(* Logix 5000 Rung export; software revision 16.04 *)

TYPE SIEDATETIME :   // Stores the date and time value
STRUCT
   Year : DINT;   // Displays module current year
   Month : DINT;   // Displays Module current month
   Day : DINT;   // Displays Module current day
   Hour : DINT;   // Displays Module current hour
   Minute : DINT;   // Displays Module current minute
   Seconds : DINT;   // Displays Module current second
END_STRUCT
END_TYPE

TYPE SIEETHERNETTYPE :   // Allows read/write Ethernet settings between the module and processor
STRUCT
   Read : BOOL;   // Enable Ethernet configuration transfer from module to processor
   Write : BOOL;   // Enable Ethernet configuration transfer from processor to module
   Config : SIEETHERNET;   // Module ethernet configurations ip, netmask and gateway
END_STRUCT
END_TYPE

TYPE SIEETHERNET :   // Stores the MVI56E-SIE IP settings
STRUCT
   IP : INT[4];   // Module IP address
   Netmask : INT[4];   // Net mask used by the Module
   Gateway : INT[4];   // Gateway used by the module
END_STRUCT
END_TYPE

TYPE SIECLOCKTYPE :   // Allows read/write of clock value between the module and processor
STRUCT
   Read : BOOL;   // Reads current time from the module
   Write : BOOL;   // Writes current time from the module
   Config : SIEDATETIME;   // Date and time configuration read or written between the module and processor
END_STRUCT
END_TYPE

ADD_ON_INSTRUCTION AOI56ESIE_OPTIONAL   (* revision 1.0 *)
// MVI56E-SIEOptional Add-On Ethernet/Clock
// Revision note:
// Release
VAR_IN_OUT
   MVI56SIEEthernet : SIEETHERNETTYPE; {required}   // MVI56E-SIE Rev2 Ethernet Settings
        .READ   // MVI56E-SIE Rev2 Ethernet Settings Enable Ethernet configuration transfer from module to processor
   MVI56SIEClock : SIECLOCKTYPE; {required}   // MVI56E-SIE Rev2 Clock Settings
   ReadEthernetMSG : MESSAGE; {required}   // Read Ethernet Settings Message
   WriteEthernetMSG : MESSAGE; {required}   // Write Ethernet Settings Message
   ReadClockMSG : MESSAGE; {required}   // Read Clock Settings Message
   WriteClockMSG : MESSAGE; {required}   // Write Clock Settings Message
END_VAR

ROUTINE Logic   (* ladder *)
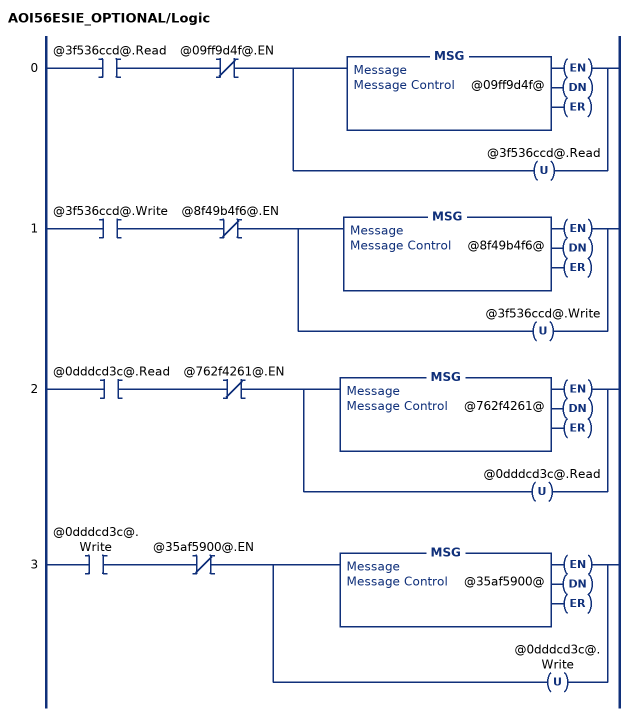
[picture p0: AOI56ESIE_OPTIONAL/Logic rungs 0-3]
   0: XIC(@3f536ccd@.Read)XIO(@09ff9d4f@.EN)[MSG(@09ff9d4f@) ,OTU(@3f536ccd@.Read) ];
   1: XIC(@3f536ccd@.Write)XIO(@8f49b4f6@.EN)[MSG(@8f49b4f6@) ,OTU(@3f536ccd@.Write) ];
   2: XIC(@0dddcd3c@.Read)XIO(@762f4261@.EN)[MSG(@762f4261@) ,OTU(@0dddcd3c@.Read) ];
   3: XIC(@0dddcd3c@.Write)XIO(@35af5900@.EN)[MSG(@35af5900@) ,OTU(@0dddcd3c@.Write) ];
END_ROUTINE
END_ADD_ON_INSTRUCTION

VAR_GLOBAL   (* controller tags *)
   MVI56ESIEETHERNET : SIEETHERNETTYPE;
   READETHERNETMSG : MESSAGE;
        MessageParameters(MessageType := CIP Generic, ConnectedFlag := 2, ConnectionPath := SIE, ServiceCode := 16#000e, ObjectType := 16#0004, TargetObject := 8, DestinationTag := MVI56ESIEETHERNET.Config)
   WRITECLOCKMSG : MESSAGE;
        MessageParameters(MessageType := CIP Generic, RequestedLength := 24, ConnectedFlag := 2, ConnectionPath := SIE, ServiceCode := 16#0010, ObjectType := 16#0004, TargetObject := 8, LocalElement := MVI56ESIECLOCK.Config)
   WRITEETHERNETMSG : MESSAGE;
        MessageParameters(MessageType := CIP Generic, RequestedLength := 24, ConnectedFlag := 2, ConnectionPath := SIE, ServiceCode := 16#0010, ObjectType := 16#0004, TargetObject := 8, LocalElement := MVI56ESIEETHERNET.Config)
   AOI56ESIE_OPTIONAL : AOI56ESIE_OPTIONAL;
   MVI56ESIECLOCK : SIECLOCKTYPE;
   READCLOCKMSG : MESSAGE;
        MessageParameters(MessageType := CIP Generic, ConnectedFlag := 2, ConnectionPath := SIE, ServiceCode := 16#000e, ObjectType := 16#0004, TargetObject := 8, AttributeNumber := 16#0020, DestinationTag := MVI56ESIECLOCK.Config)
END_VAR

PROGRAM MainProgram

ROUTINE MainRoutine   (* ladder *)
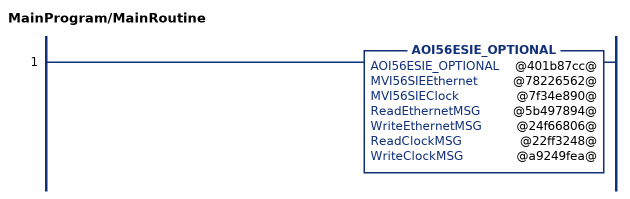
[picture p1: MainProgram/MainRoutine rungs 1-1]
   1: AOI56ESIE_OPTIONAL(@401b87cc@,@78226562@,@7f34e890@,@5b497894@,@24f66806@,@22ff3248@,@a9249fea@);
END_ROUTINE
END_PROGRAM
